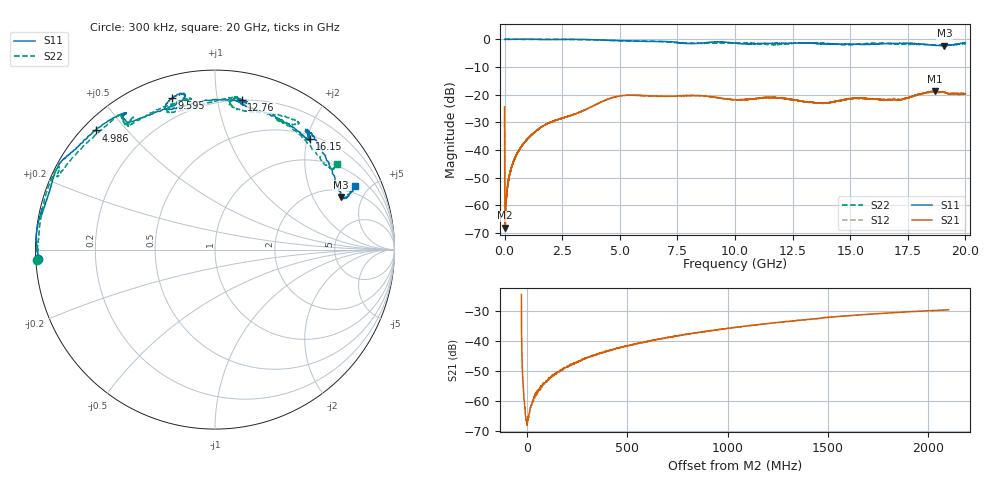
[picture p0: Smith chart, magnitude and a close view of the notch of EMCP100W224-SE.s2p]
!{EMCP100W224}
!Johanson Technology Inc.
!www.johansontechnology.com
!Test Board Conditions:
!Substrate Type  RO4350B
!Substrate Thickness  10 mil
!Substrate Dk  3.66
!TL Type: GCPW
!TL Trace Width  20 mil
!TL Gap  10 mil
!PART MODE SINGLE ENDED (AKA BYPASS)
!DUT TOPOLOGY	SERIES-SHUNT
# MHz S  dB  R 50
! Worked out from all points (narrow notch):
!   20001 points, 300 kHz to 20 GHz, reference 50 ohm
!   highest |S21| = -18.82 dB at 18.68 GHz (marker M1); lowest = -68.0 dB at 29.3 MHz (marker M2)
!   notch at M2: 46.5 dB deep, 351 MHz wide at half that depth
!   lowest |S11| = -2.4 dB at 19.09 GHz (marker M3), VSWR 7.32, Z = 120 + j167 ohm
!   |S11| at or under -10 dB: nowhere
!   |S22| runs from -2.3 to 0.0 dB; largest |S21 - S12| = 0.0061
!   S11 on the Smith chart (normalised r, x): 300 kHz: 0.01, -0.03; 4.986 GHz: 0.04, +0.41; 9.595 GHz: 0.10, +0.75; 12.76 GHz: 0.20, +1.18; 16.15 GHz: 0.56, +2.04; 20 GHz: 1.56, +4.08
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0.3  -0.12 -176.9  -24.46 -85.5  -24.50 -85.8  -0.07 -176.5
29.3  -0.10 180.0  -68.03 -3.5  -67.55 2.2  -0.06 -180.0
106.298  -0.10 179.9  -54.41 70.3  -54.40 62.4  -0.06 179.8
388.294  -0.08 179.2  -44.26 76.6  -44.20 77.1  -0.07 179.4
991.285  -0.01 174.2  -36.06 75.4  -36.04 75.6  -0.13 176.2
2301.265  -0.18 159.0  -29.07 56.9  -29.08 57.2  -0.07 154.2
3334.25  -0.11 150.3  -26.12 50.0  -26.09 49.9  -0.24 154.1
4986.225  -0.54 135.1  -20.55 21.7  -20.48 21.8  -0.65 139.1
6667.2  -0.84 124.0  -20.59 -13.0  -20.66 -12.4  -0.83 125.1
8302.175  -1.59 106.5  -20.38 -31.5  -20.41 -31.5  -1.53 123.8
9595.156  -1.16 105.8  -21.56 -45.2  -21.62 -45.9  -1.44 99.9
10000.15  -1.46 109.2  -21.88 -45.6  -22.03 -45.9  -1.38 99.4
11266.13  -1.57 89.6  -21.21 -53.4  -21.06 -53.6  -1.85 108.8
12758.11  -1.44 79.9  -22.19 -68.7  -22.24 -68.6  -1.41 83.9
13334.1  -1.47 81.2  -22.82 -68.5  -22.81 -68.1  -1.34 81.6
14595.08  -1.77 68.7  -22.20 -68.3  -22.00 -68.4  -1.96 82.3
16151.06  -1.80 49.6  -21.75 -80.9  -21.70 -79.1  -1.45 57.6
16667.05  -1.62 51.7  -22.00 -78.6  -21.77 -77.8  -1.60 57.0
17644.03  -1.56 48.9  -20.86 -75.0  -20.89 -76.4  -1.91 64.0
18680.02  -2.23 28.4  -18.82 -91.9  -19.11 -91.7  -2.15 46.6
19086.01  -2.39 22.7  -19.21 -98.9  -19.25 -96.8  -2.23 38.5
20000  -1.36 24.3  -19.75 -95.7  -19.35 -97.0  -1.63 35.1
